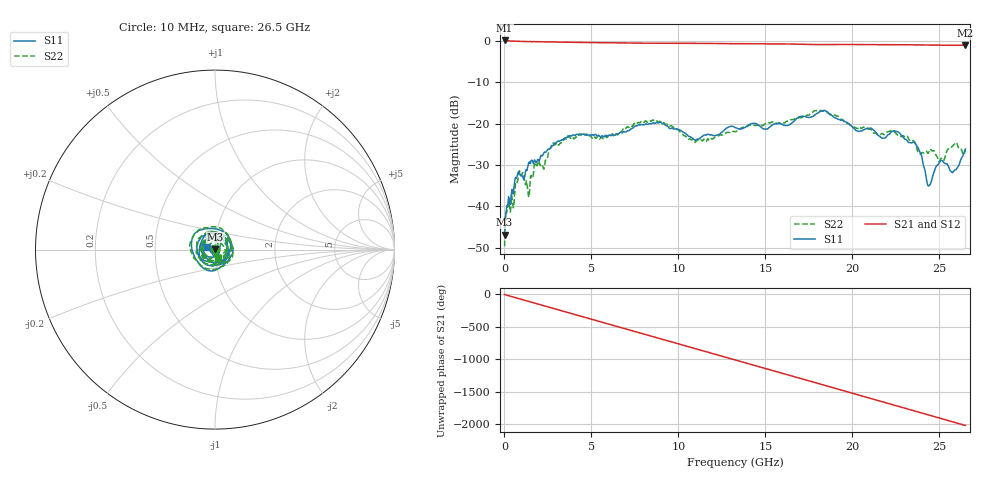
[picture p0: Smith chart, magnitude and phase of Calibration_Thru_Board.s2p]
!Agilent Technologies,N5222A,MY51421700,A.10.00.00
!Agilent N5222A: A.10.00.00
!Date: Thursday, April 02, 2015 22:15:09
!Correction: S11(Full 2 Port(1,2))
!S21(Full 2 Port(1,2))
!S12(Full 2 Port(1,2))
!S22(Full 2 Port(1,2))
!S2P File: Measurements: S11, S21, S12, S22:
# Hz S  dB  R 50
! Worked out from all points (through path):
!   801 points, 10 MHz to 26.5 GHz, reference 50 ohm
!   highest |S21| = 0.06 dB at 10 MHz (marker M1); lowest = -1.1 dB at 26.5 GHz (marker M2)
!   group delay of S21, straight-line fit = 211 ps
!   lowest |S11| = -46.8 dB at 10 MHz (marker M3), VSWR 1.01, Z = 50.2 + j0.411 ohm
!   |S11| at or under -10 dB: start of sweep to end of sweep
!   |S22| runs from -49.6 to -16.8 dB; largest |S21 - S12| = 0.0085
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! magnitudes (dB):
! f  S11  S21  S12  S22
! 10 MHz  -46.8  0.1  0.0  -49.6
! 175.6 MHz  -40.2  0.0  -0.1  -39.6
! 440.5 MHz  -35.9  -0.1  -0.1  -37.9
! 705.4 MHz  -33.1  -0.1  -0.2  -34.4
! 937.1 MHz  -32.6  -0.2  -0.2  -32.2
! 1.335 GHz  -30.5  -0.2  -0.3  -35.8
! 1.831 GHz  -29.5  -0.2  -0.3  -30.0
! 2.328 GHz  -26.9  -0.3  -0.3  -29.5
! 2.725 GHz  -25.3  -0.3  -0.4  -25.4
! 4.447 GHz  -22.6  -0.4  -0.5  -22.6
! 8.851 GHz  -19.9  -0.6  -0.7  -19.6
! 10.9 GHz  -23.9  -0.6  -0.7  -24.2
! 13.26 GHz  -21.0  -0.7  -0.8  -21.9
! 17.69 GHz  -18.3  -0.9  -1.0  -17.3
! 18.45 GHz  -17.0  -0.9  -1.0  -17.1
! 20.31 GHz  -21.8  -0.9  -1.0  -21.2
! 22.1 GHz  -22.6  -1.0  -1.0  -21.9
! 23.65 GHz  -25.1  -1.0  -1.1  -25.0
! 24.41 GHz  -35.0  -1.0  -1.1  -26.7
! 25.01 GHz  -29.4  -1.1  -1.1  -29.1
! 25.84 GHz  -31.4  -1.1  -1.2  -25.1
! 26.5 GHz  -26.1  -1.1  -1.2  -26.4
